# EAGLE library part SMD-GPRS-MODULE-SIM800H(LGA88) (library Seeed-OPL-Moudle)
317040001
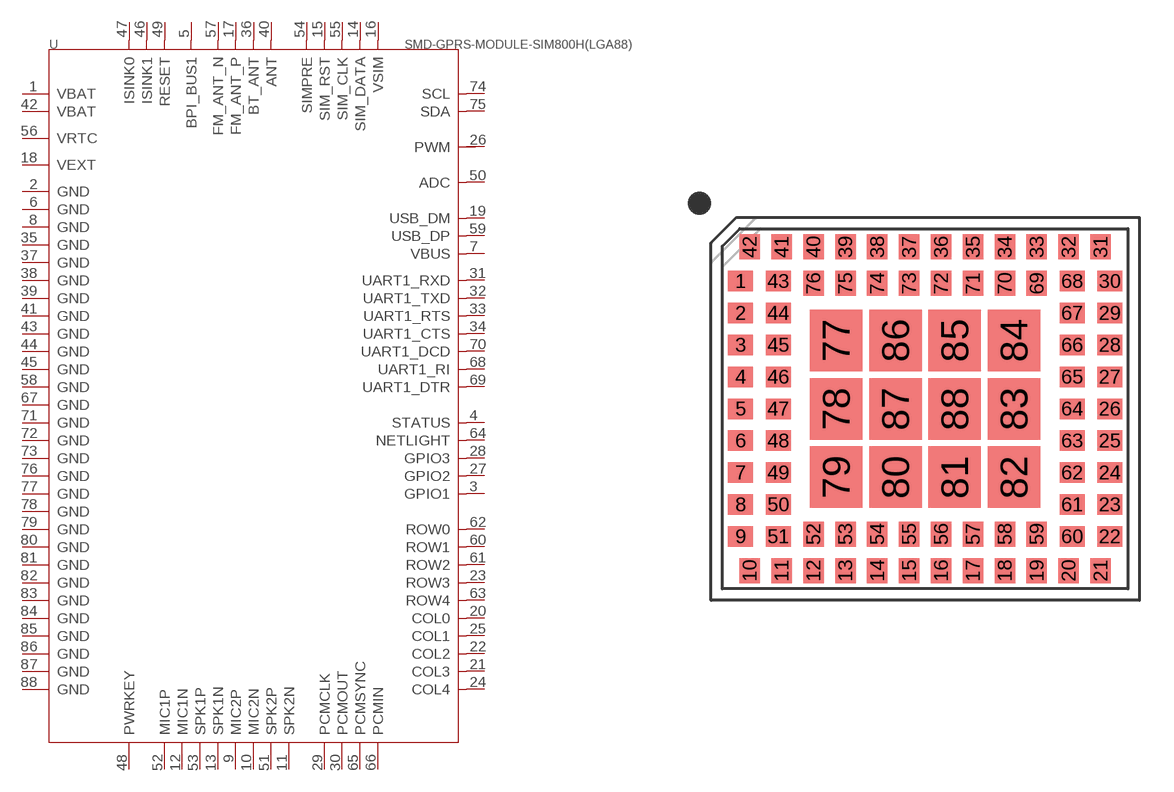
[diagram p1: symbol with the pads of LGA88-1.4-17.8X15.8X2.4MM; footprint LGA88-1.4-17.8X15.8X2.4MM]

Designator prefix U

## SMD-GPRS-MODULE-SIM800H(LGA88)-SIM800H (MPN: SIM800H; VALUE: SIM800H)  [LGA88-1.4-17.8X15.8X2.4MM]
1  VBAT
2  GND
3  GPIO1
4  STATUS
5  BPI_BUS1
6  GND
7  VBUS
8  GND
9  MIC2P
10  MIC2N
11  SPK2N
12  MIC1N
13  SPK1N
14  SIM_DATA
15  SIM_RST
16  VSIM
17  FM_ANT_P
18  VEXT
19  USB_DM
20  COL0
21  COL3
22  COL2
23  ROW3
24  COL4
25  COL1
26  PWM
27  GPIO2
28  GPIO3
29  PCMCLK
30  PCMOUT
31  UART1_RXD
32  UART1_TXD
33  UART1_RTS
34  UART1_CTS
35  GND
36  BT_ANT
37  GND
38  GND
39  GND
40  ANT
41  GND
42  VBAT
43  GND
44  GND
45  GND
46  ISINK1
47  ISINK0
48  PWRKEY
49  RESET
50  ADC
51  SPK2P
52  MIC1P
53  SPK1P
54  SIMPRE
55  SIM_CLK
56  VRTC
57  FM_ANT_N
58  GND
59  USB_DP
60  ROW1
61  ROW2
62  ROW0
63  ROW4
64  NETLIGHT
65  PCMSYNC
66  PCMIN
67  GND
68  UART1_RI
69  UART1_DTR
70  UART1_DCD
71  GND
72  GND
73  GND
74  SCL
75  SDA
76  GND
77  GND
78  GND
79  GND
80  GND
81  GND
82  GND
83  GND
84  GND
85  GND
86  GND
87  GND
88  GND

## Footprint LGA88-1.4-17.8X15.8X2.4MM (pad centres in mm)
smd 1.1 x 0.9: 1 -8.1,5.6; 2 -8.1,4.2; 3 -8.1,2.8; 4 -8.1,1.4; 5 -8.1,0; 6 -8.1,-1.4; 7 -8.1,-2.8; 8 -8.1,-4.2; 9 -8.1,-5.6; 22 8.1,-5.6; 23 8.1,-4.2; 24 8.1,-2.8; 25 8.1,-1.4; 26 8.1,0; 27 8.1,1.4; 28 8.1,2.8; 29 8.1,4.2; 30 8.1,5.6; 43 -6.45,5.6; 44 -6.45,4.2; 45 -6.45,2.8; 46 -6.45,1.4; 47 -6.45,0; 48 -6.45,-1.4; 49 -6.45,-2.8; 50 -6.45,-4.2; 51 -6.45,-5.6; 60 6.45,-5.6; 61 6.45,-4.2; 62 6.45,-2.8; 63 6.45,-1.4; 64 6.45,0; 65 6.45,1.4; 66 6.45,2.8; 67 6.45,4.2; 68 6.45,5.6
smd 0.9 x 1.1: 10 -7.7,-7.1; 11 -6.3,-7.1; 12 -4.9,-7.1; 13 -3.5,-7.1; 14 -2.1,-7.1; 15 -0.7,-7.1; 16 0.7,-7.1; 17 2.1,-7.1; 18 3.5,-7.1; 19 4.9,-7.1; 20 6.3,-7.1; 21 7.7,-7.1; 31 7.7,7.1; 32 6.3,7.1; 33 4.9,7.1; 34 3.5,7.1; 35 2.1,7.1; 36 0.7,7.1; 37 -0.7,7.1; 38 -2.1,7.1; 39 -3.5,7.1; 40 -4.9,7.1; 41 -6.3,7.1; 42 -7.7,7.1; 52 -4.9,-5.5; 53 -3.5,-5.5; 54 -2.1,-5.5; 55 -0.7,-5.5; 56 0.7,-5.5; 57 2.1,-5.5; 58 3.5,-5.5; 59 4.9,-5.5; 69 4.9,5.5; 70 3.5,5.5; 71 2.1,5.5; 72 0.7,5.5; 73 -0.7,5.5; 74 -2.1,5.5; 75 -3.5,5.5; 76 -4.9,5.5
smd 2.3 x 2.7: 77 -3.9,3; 78 -3.9,0; 79 -3.9,-3; 80 -1.3,-3; 81 1.3,-3; 82 3.9,-3; 83 3.9,0; 84 3.9,3; 85 1.3,3; 86 -1.3,3; 87 -1.3,0; 88 1.3,0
